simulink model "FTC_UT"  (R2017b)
settings: Solver=FixedStepDiscrete  StartTime=0.0  StopTime=10.0  FixedStep=0.01  RelTol=1e-3  EnableMultiTasking=on
libraries: AIWAYS_Powertrain_BMS_lib x19

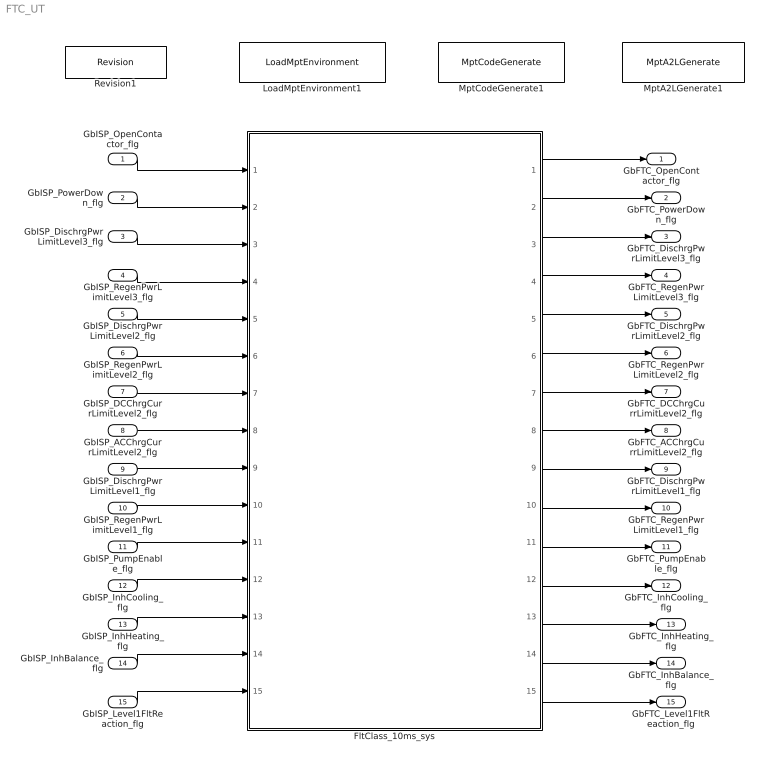
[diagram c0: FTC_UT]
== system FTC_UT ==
  GbISP_OpenContactor_flg : Inport
  GbISP_PowerDown_flg : Inport  Port=2
  GbISP_DischrgPwrLimitLevel3_flg : Inport  Port=3
  GbISP_RegenPwrLimitLevel3_flg : Inport  Port=4
  GbISP_DischrgPwrLimitLevel2_flg : Inport  Port=5
  GbISP_RegenPwrLimitLevel2_flg : Inport  Port=6
  GbISP_DCChrgCurrLimitLevel2_flg : Inport  Port=7
  GbISP_ACChrgCurrLimitLevel2_flg : Inport  Port=8
  GbISP_DischrgPwrLimitLevel1_flg : Inport  Port=9
  GbISP_RegenPwrLimitLevel1_flg : Inport  Port=10
  GbISP_PumpEnable_flg : Inport  Port=11
  GbISP_InhCooling_flg : Inport  Port=12
  GbISP_InhHeating_flg : Inport  Port=13
  GbISP_InhBalance_flg : Inport  Port=14
  GbISP_Level1FltReaction_flg : Inport  Port=15
  FltClass_10ms_sys : Subsystem
  LoadMptEnvironment1 : AIWAYS_Powertrain_BMS_lib/Config/LoadMptEnvironment  ProjectName=Comm  SuppierID=NewPlatformUAES
  MptA2LGenerate1 : AIWAYS_Powertrain_BMS_lib/Config/MptA2LGenerate  SystemSampleTime=-1
  MptCodeGenerate1 : AIWAYS_Powertrain_BMS_lib/Config/MptCodeGenerate  SystemSampleTime=-1
  Revision1 : AIWAYS_Powertrain_BMS_lib/Config/Revision  curVersion='M100C100'  newVersion='M100C100'
  GbFTC_OpenContactor_flg : Outport
  GbFTC_PowerDown_flg : Outport  Port=2
  GbFTC_DischrgPwrLimitLevel3_flg : Outport  Port=3
  GbFTC_RegenPwrLimitLevel3_flg : Outport  Port=4
  GbFTC_DischrgPwrLimitLevel2_flg : Outport  Port=5
  GbFTC_RegenPwrLimitLevel2_flg : Outport  Port=6
  GbFTC_DCChrgCurrLimitLevel2_flg : Outport  Port=7
  GbFTC_ACChrgCurrLimitLevel2_flg : Outport  Port=8
  GbFTC_DischrgPwrLimitLevel1_flg : Outport  Port=9
  GbFTC_RegenPwrLimitLevel1_flg : Outport  Port=10
  GbFTC_PumpEnable_flg : Outport  Port=11
  GbFTC_InhCooling_flg : Outport  Port=12
  GbFTC_InhHeating_flg : Outport  Port=13
  GbFTC_InhBalance_flg : Outport  Port=14
  GbFTC_Level1FltReaction_flg : Outport  Port=15
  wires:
  FltClass_10ms_sys/1(GbFTC_OpenContactor_flg) -> GbFTC_OpenContactor_flg/1
  GbISP_DischrgPwrLimitLevel3_flg/1 -> FltClass_10ms_sys/3(GbISP_DischrgPwrLimitLevel3_flg)
  GbISP_RegenPwrLimitLevel1_flg/1 -> FltClass_10ms_sys/10(GbISP_RegenPwrLimitLevel1_flg)
  GbISP_DCChrgCurrLimitLevel2_flg/1 -> FltClass_10ms_sys/7(GbISP_DCChrgCurrLimitLevel2_flg)
  FltClass_10ms_sys/14(GbFTC_InhBalance_flg) -> GbFTC_InhBalance_flg/1
  GbISP_InhBalance_flg/1 -> FltClass_10ms_sys/14(GbISP_InhBalance_flg)
  FltClass_10ms_sys/2(GbFTC_PowerDown_flg) -> GbFTC_PowerDown_flg/1
  GbISP_RegenPwrLimitLevel3_flg/1 -> FltClass_10ms_sys/4(GbISP_RegenPwrLimitLevel3_flg)
  FltClass_10ms_sys/10(GbFTC_RegenPwrLimitLevel1_flg) -> GbFTC_RegenPwrLimitLevel1_flg/1
  FltClass_10ms_sys/15(GbFTC_Level1FltReaction_flg) -> GbFTC_Level1FltReaction_flg/1
  GbISP_OpenContactor_flg/1 -> FltClass_10ms_sys/1(GbISP_OpenContactor_flg)
  FltClass_10ms_sys/12(GbFTC_InhCooling_flg) -> GbFTC_InhCooling_flg/1
  FltClass_10ms_sys/13(GbFTC_InhHeating_flg) -> GbFTC_InhHeating_flg/1
  FltClass_10ms_sys/3(GbFTC_DischrgPwrLimitLevel3_flg) -> GbFTC_DischrgPwrLimitLevel3_flg/1
  FltClass_10ms_sys/7(GbFTC_DCChrgCurrLimitLevel2_flg) -> GbFTC_DCChrgCurrLimitLevel2_flg/1
  GbISP_DischrgPwrLimitLevel1_flg/1 -> FltClass_10ms_sys/9(GbISP_DischrgPwrLimitLevel1_flg)
  GbISP_PumpEnable_flg/1 -> FltClass_10ms_sys/11(GbISP_PumpEnable_flg)
  FltClass_10ms_sys/9(GbFTC_DischrgPwrLimitLevel1_flg) -> GbFTC_DischrgPwrLimitLevel1_flg/1
  FltClass_10ms_sys/11(GbFTC_PumpEnable_flg) -> GbFTC_PumpEnable_flg/1
  GbISP_RegenPwrLimitLevel2_flg/1 -> FltClass_10ms_sys/6(GbISP_RegenPwrLimitLevel2_flg)
  GbISP_Level1FltReaction_flg/1 -> FltClass_10ms_sys/15(GbISP_Level1FltReaction_flg)
  GbISP_PowerDown_flg/1 -> FltClass_10ms_sys/2(GbISP_PowerDown_flg)
  FltClass_10ms_sys/6(GbFTC_RegenPwrLimitLevel2_flg) -> GbFTC_RegenPwrLimitLevel2_flg/1
  GbISP_DischrgPwrLimitLevel2_flg/1 -> FltClass_10ms_sys/5(GbISP_DischrgPwrLimitLevel2_flg)
  GbISP_InhCooling_flg/1 -> FltClass_10ms_sys/12(GbISP_InhCooling_flg)
  FltClass_10ms_sys/5(GbFTC_DischrgPwrLimitLevel2_flg) -> GbFTC_DischrgPwrLimitLevel2_flg/1
  FltClass_10ms_sys/4(GbFTC_RegenPwrLimitLevel3_flg) -> GbFTC_RegenPwrLimitLevel3_flg/1
  GbISP_InhHeating_flg/1 -> FltClass_10ms_sys/13(GbISP_InhHeating_flg)
  GbISP_ACChrgCurrLimitLevel2_flg/1 -> FltClass_10ms_sys/8(GbISP_ACChrgCurrLimitLevel2_flg)
  FltClass_10ms_sys/8(GbFTC_ACChrgCurrLimitLevel2_flg) -> GbFTC_ACChrgCurrLimitLevel2_flg/1

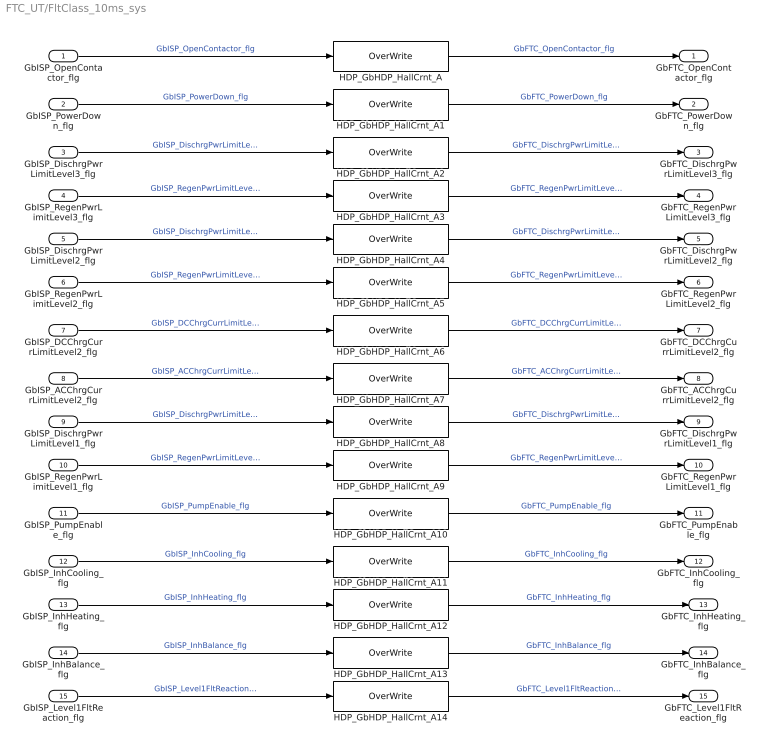
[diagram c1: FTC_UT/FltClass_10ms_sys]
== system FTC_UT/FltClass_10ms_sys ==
  GbISP_OpenContactor_flg : Inport
  GbISP_PowerDown_flg : Inport  Port=2
  GbISP_DischrgPwrLimitLevel3_flg : Inport  Port=3
  GbISP_RegenPwrLimitLevel3_flg : Inport  Port=4
  GbISP_DischrgPwrLimitLevel2_flg : Inport  Port=5
  GbISP_RegenPwrLimitLevel2_flg : Inport  Port=6
  GbISP_DCChrgCurrLimitLevel2_flg : Inport  Port=7
  GbISP_ACChrgCurrLimitLevel2_flg : Inport  Port=8
  GbISP_DischrgPwrLimitLevel1_flg : Inport  Port=9
  GbISP_RegenPwrLimitLevel1_flg : Inport  Port=10
  GbISP_PumpEnable_flg : Inport  Port=11
  GbISP_InhCooling_flg : Inport  Port=12
  GbISP_InhHeating_flg : Inport  Port=13
  GbISP_InhBalance_flg : Inport  Port=14
  GbISP_Level1FltReaction_flg : Inport  Port=15
  HDP_GbHDP_HallCrnt_A : AIWAYS_Powertrain_BMS_lib/Signals/OverWrite  OverWrite_Value=CbFTC_OpenContactorOvr_flg  OverWrite_flag=CbFTC_OpenContactorOvrSwt_flg
  HDP_GbHDP_HallCrnt_A1 : AIWAYS_Powertrain_BMS_lib/Signals/OverWrite  OverWrite_Value=CbFTC_PowerDownOvr_flg  OverWrite_flag=CbFTC_PowerDownOvrSwt_flg
  HDP_GbHDP_HallCrnt_A10 : AIWAYS_Powertrain_BMS_lib/Signals/OverWrite  OverWrite_Value=CbFTC_PumpEnableOvr_flg  OverWrite_flag=CbFTC_PumpEnableOvrSwt_flg
  HDP_GbHDP_HallCrnt_A11 : AIWAYS_Powertrain_BMS_lib/Signals/OverWrite  OverWrite_Value=CbFTC_InhCoolingOvr_flg  OverWrite_flag=CbFTC_InhCoolingOvrSwt_flg
  HDP_GbHDP_HallCrnt_A12 : AIWAYS_Powertrain_BMS_lib/Signals/OverWrite  OverWrite_Value=CbFTC_InhHeatingOvr_flg  OverWrite_flag=CbFTC_InhHeatingOvrSwt_flg
  HDP_GbHDP_HallCrnt_A13 : AIWAYS_Powertrain_BMS_lib/Signals/OverWrite  OverWrite_Value=CbFTC_InhBalanceOvr_flg  OverWrite_flag=CbFTC_InhBalanceOvrSwt_flg
  HDP_GbHDP_HallCrnt_A14 : AIWAYS_Powertrain_BMS_lib/Signals/OverWrite  OverWrite_Value=CbFTC_Level1FltReactionOvr_flg  OverWrite_flag=CbFTC_Level1FltReactionOvrSwt_flg
  HDP_GbHDP_HallCrnt_A2 : AIWAYS_Powertrain_BMS_lib/Signals/OverWrite  OverWrite_Value=CbFTC_DischrgPwrLimitLevel3Ovr_flg  OverWrite_flag=CbFTC_DischrgPwrLimitLevel3OvrSwt_flg
  HDP_GbHDP_HallCrnt_A3 : AIWAYS_Powertrain_BMS_lib/Signals/OverWrite  OverWrite_Value=CbFTC_RegenPwrLimitLevel3Ovr_flg  OverWrite_flag=CbFTC_RegenPwrLimitLevel3OvrSwt_flg
  HDP_GbHDP_HallCrnt_A4 : AIWAYS_Powertrain_BMS_lib/Signals/OverWrite  OverWrite_Value=CbFTC_DischrgPwrLimitLevel2Ovr_flg  OverWrite_flag=CbFTC_DischrgPwrLimitLevel2OvrSwt_flg
  HDP_GbHDP_HallCrnt_A5 : AIWAYS_Powertrain_BMS_lib/Signals/OverWrite  OverWrite_Value=CbFTC_RegenPwrLimitLevel2Ovr_flg  OverWrite_flag=CbFTC_RegenPwrLimitLevel2OvrSwt_flg
  HDP_GbHDP_HallCrnt_A6 : AIWAYS_Powertrain_BMS_lib/Signals/OverWrite  OverWrite_Value=CbFTC_DCChrgCurrLimitLevel2Ovr_flg  OverWrite_flag=CbFTC_DCChrgCurrLimitLevel2OvrSwt_flg
  HDP_GbHDP_HallCrnt_A7 : AIWAYS_Powertrain_BMS_lib/Signals/OverWrite  OverWrite_Value=CbFTC_ACChrgCurrLimitLevel2Ovr_flg  OverWrite_flag=CbFTC_ACChrgCurrLimitLevel2OvrSwt_flg
  HDP_GbHDP_HallCrnt_A8 : AIWAYS_Powertrain_BMS_lib/Signals/OverWrite  OverWrite_Value=CbFTC_DischrgPwrLimitLevel1Ovr_flg  OverWrite_flag=CbFTC_DischrgPwrLimitLevel1OvrSwt_flg
  HDP_GbHDP_HallCrnt_A9 : AIWAYS_Powertrain_BMS_lib/Signals/OverWrite  OverWrite_Value=CbFTC_RegenPwrLimitLevel1Ovr_flg  OverWrite_flag=CbFTC_RegenPwrLimitLevel1OvrSwt_flg
  GbFTC_OpenContactor_flg : Outport
  GbFTC_PowerDown_flg : Outport  Port=2
  GbFTC_DischrgPwrLimitLevel3_flg : Outport  Port=3
  GbFTC_RegenPwrLimitLevel3_flg : Outport  Port=4
  GbFTC_DischrgPwrLimitLevel2_flg : Outport  Port=5
  GbFTC_RegenPwrLimitLevel2_flg : Outport  Port=6
  GbFTC_DCChrgCurrLimitLevel2_flg : Outport  Port=7
  GbFTC_ACChrgCurrLimitLevel2_flg : Outport  Port=8
  GbFTC_DischrgPwrLimitLevel1_flg : Outport  Port=9
  GbFTC_RegenPwrLimitLevel1_flg : Outport  Port=10
  GbFTC_PumpEnable_flg : Outport  Port=11
  GbFTC_InhCooling_flg : Outport  Port=12
  GbFTC_InhHeating_flg : Outport  Port=13
  GbFTC_InhBalance_flg : Outport  Port=14
  GbFTC_Level1FltReaction_flg : Outport  Port=15
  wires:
  HDP_GbHDP_HallCrnt_A/1 -> GbFTC_OpenContactor_flg/1  "GbFTC_OpenContactor_flg"
  GbISP_OpenContactor_flg/1 -> HDP_GbHDP_HallCrnt_A/1  "GbISP_OpenContactor_flg"
  GbISP_PowerDown_flg/1 -> HDP_GbHDP_HallCrnt_A1/1  "GbISP_PowerDown_flg"
  HDP_GbHDP_HallCrnt_A1/1 -> GbFTC_PowerDown_flg/1  "GbFTC_PowerDown_flg"
  GbISP_DischrgPwrLimitLevel3_flg/1 -> HDP_GbHDP_HallCrnt_A2/1  "GbISP_DischrgPwrLimitLevel3_flg"
  HDP_GbHDP_HallCrnt_A2/1 -> GbFTC_DischrgPwrLimitLevel3_flg/1  "GbFTC_DischrgPwrLimitLevel3_flg"
  GbISP_RegenPwrLimitLevel3_flg/1 -> HDP_GbHDP_HallCrnt_A3/1  "GbISP_RegenPwrLimitLevel3_flg"
  HDP_GbHDP_HallCrnt_A3/1 -> GbFTC_RegenPwrLimitLevel3_flg/1  "GbFTC_RegenPwrLimitLevel3_flg"
  GbISP_DischrgPwrLimitLevel2_flg/1 -> HDP_GbHDP_HallCrnt_A4/1  "GbISP_DischrgPwrLimitLevel2_flg"
  HDP_GbHDP_HallCrnt_A4/1 -> GbFTC_DischrgPwrLimitLevel2_flg/1  "GbFTC_DischrgPwrLimitLevel2_flg"
  GbISP_RegenPwrLimitLevel2_flg/1 -> HDP_GbHDP_HallCrnt_A5/1  "GbISP_RegenPwrLimitLevel2_flg"
  HDP_GbHDP_HallCrnt_A5/1 -> GbFTC_RegenPwrLimitLevel2_flg/1  "GbFTC_RegenPwrLimitLevel2_flg"
  GbISP_DCChrgCurrLimitLevel2_flg/1 -> HDP_GbHDP_HallCrnt_A6/1  "GbISP_DCChrgCurrLimitLevel2_flg"
  HDP_GbHDP_HallCrnt_A6/1 -> GbFTC_DCChrgCurrLimitLevel2_flg/1  "GbFTC_DCChrgCurrLimitLevel2_flg"
  GbISP_ACChrgCurrLimitLevel2_flg/1 -> HDP_GbHDP_HallCrnt_A7/1  "GbISP_ACChrgCurrLimitLevel2_flg"
  GbISP_DischrgPwrLimitLevel1_flg/1 -> HDP_GbHDP_HallCrnt_A8/1  "GbISP_DischrgPwrLimitLevel1_flg"
  GbISP_RegenPwrLimitLevel1_flg/1 -> HDP_GbHDP_HallCrnt_A9/1  "GbISP_RegenPwrLimitLevel1_flg"
  GbISP_PumpEnable_flg/1 -> HDP_GbHDP_HallCrnt_A10/1  "GbISP_PumpEnable_flg"
  GbISP_InhCooling_flg/1 -> HDP_GbHDP_HallCrnt_A11/1  "GbISP_InhCooling_flg"
  GbISP_InhHeating_flg/1 -> HDP_GbHDP_HallCrnt_A12/1  "GbISP_InhHeating_flg"
  GbISP_InhBalance_flg/1 -> HDP_GbHDP_HallCrnt_A13/1  "GbISP_InhBalance_flg"
  GbISP_Level1FltReaction_flg/1 -> HDP_GbHDP_HallCrnt_A14/1  "GbISP_Level1FltReaction_flg"
  HDP_GbHDP_HallCrnt_A7/1 -> GbFTC_ACChrgCurrLimitLevel2_flg/1  "GbFTC_ACChrgCurrLimitLevel2_flg"
  HDP_GbHDP_HallCrnt_A8/1 -> GbFTC_DischrgPwrLimitLevel1_flg/1  "GbFTC_DischrgPwrLimitLevel1_flg"
  HDP_GbHDP_HallCrnt_A9/1 -> GbFTC_RegenPwrLimitLevel1_flg/1  "GbFTC_RegenPwrLimitLevel1_flg"
  HDP_GbHDP_HallCrnt_A10/1 -> GbFTC_PumpEnable_flg/1  "GbFTC_PumpEnable_flg"
  HDP_GbHDP_HallCrnt_A11/1 -> GbFTC_InhCooling_flg/1  "GbFTC_InhCooling_flg"
  HDP_GbHDP_HallCrnt_A12/1 -> GbFTC_InhHeating_flg/1  "GbFTC_InhHeating_flg"
  HDP_GbHDP_HallCrnt_A13/1 -> GbFTC_InhBalance_flg/1  "GbFTC_InhBalance_flg"
  HDP_GbHDP_HallCrnt_A14/1 -> GbFTC_Level1FltReaction_flg/1  "GbFTC_Level1FltReaction_flg"
